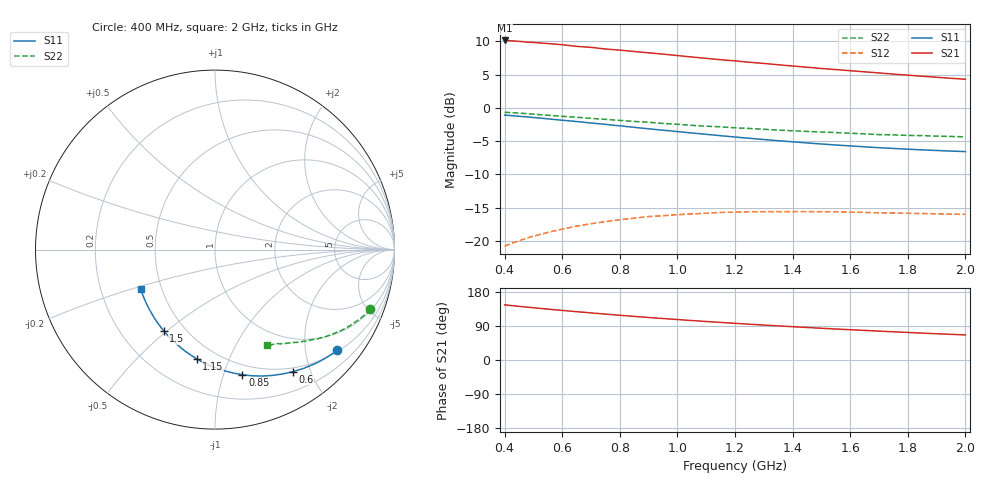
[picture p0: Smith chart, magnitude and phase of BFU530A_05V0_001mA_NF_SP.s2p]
! Filename:  P:\Prog\Test\Noise\ATS_data\Testdata_Net\06 Compressed Noise after Statistics\BFU530A_APG2013_33_A05_05p0V_001mA_SP_CM01_D.sf
! Date/Time: Tue 16/Apr/2013 15:10:54
! BFU530A_APG2013_33_A05_05p0V_1to25mA_NF_CM01_Bias1_R.sf
! Noise Parameter Data File
! BFU530A_APG2013_33_A05_05p0V_1to25mA_NF_CM01
! Date/time: Fri Apr 12 15:27:54 2013
! freq range =  0.4000 to  2.0000 GHz, 37 points
! bias range =  1.0000 to 25.0000 mA, 8 points
! bias supplies used: 1 1 0 0 0 0
! VAR bias_mode= 1  ! Specify V_out, I_out
! VAR bias_var = 1  ! Bias variable = I_out
! VAR V_out= 5.001000
! VAR I_out= 1.000000
! VAR V_in= 0.783300
! VAR I_in= 0.010301
! Device data file deembeded for feedlines and parallel
! Original file: \06 Compressed Noise after Statistics\BFU530A_APG2013_33_A05_05p0V_001mA_SP_CM01_R.sf
! Feed-files: PR017V01_150413_Feed1.s2p, PR017V01_150413_Feed2.s2p
! Parallel-file: PR017V01_150413_Par.s2p
# MHz S MA R 50
!  Freq-MHz  S11-mag  S11-arg  S21-mag  S21-arg  S12-mag  S12-arg  S22-mag  S22-arg
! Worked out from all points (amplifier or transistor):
!   37 points, 400 MHz to 2 GHz, reference 50 ohm
!   highest |S21| = 10.1 dB at 400 MHz (marker M1)
!   |S21| within 3 dB of that: start of sweep to 1.18 GHz
!   unconditionally stable (mu >= 1): nowhere
!   at 500 MHz: K = 0.23, MSG = 14.5 dB, |S12| = -19.3 dB
!   at 1.1 GHz: K = 0.48, MSG = 11.6 dB, |S12| = -15.8 dB
!   at 2 GHz: K = 0.88, MSG = 10.1 dB, |S12| = -16.0 dB
!   lowest NFmin = 0.41 dB at 433 MHz
!   S11 on the Smith chart (normalised r, x): 400 MHz: 0.53, -2.70; 600 MHz: 0.45, -1.74; 850 MHz: 0.41, -1.16; 1.15 GHz: 0.39, -0.77; 1.5 GHz: 0.38, -0.49; 2 GHz: 0.38, -0.22
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400  0.8821 -39.4  3.205 145.5  0.09142 65.2  0.9266 -20.9
420  0.8752 -41.4  3.193 143.8  0.0951 64.1  0.9205 -21.9
440  0.8679 -43.2  3.168 142.3  0.09865 63.0  0.915 -22.7
480  0.8538 -46.7  3.109 139.4  0.1054 61.0  0.9026 -24.5
500  0.8459 -48.6  3.097 137.9  0.1086 60.0  0.8965 -25.3
550  0.8265 -53.1  3.038 134.3  0.1159 57.6  0.8795 -27.4
600  0.8068 -57.4  2.979 130.8  0.1228 55.4  0.8639 -29.3
650  0.7891 -61.5  2.893 127.5  0.1293 53.3  0.8497 -31.0
700  0.7692 -65.8  2.845 124.2  0.1346 51.2  0.8335 -32.8
750  0.7516 -69.6  2.764 121.1  0.1399 49.4  0.8189 -34.4
800  0.7324 -73.7  2.712 118.1  0.1444 47.6  0.8044 -36.0
850  0.7136 -77.6  2.648 115.0  0.1484 45.9  0.7903 -37.5
950  0.6788 -85.2  2.531 109.4  0.1548 42.9  0.7632 -40.4
1050  0.6471 -92.3  2.408 104.1  0.1597 40.3  0.7386 -42.8
1150  0.6176 -99.4  2.299 99.2  0.1638 38.0  0.7197 -45.1
1200  0.6035 -102.8  2.25 96.8  0.1644 37.0  0.7077 -46.3
1350  0.5663 -112.7  2.106 90.0  0.166 34.7  0.6799 -49.5
1500  0.5351 -122.3  1.975 83.8  0.166 33.0  0.6579 -52.5
1650  0.5094 -131.5  1.864 78.1  0.1639 32.5  0.6378 -55.4
1750  0.4955 -137.5  1.792 74.4  0.1623 32.6  0.626 -57.1
1850  0.4834 -143.2  1.728 71.0  0.1608 33.0  0.6182 -59.0
2000  0.4692 -151.8  1.638 66.1  0.1584 34.6  0.6052 -61.7
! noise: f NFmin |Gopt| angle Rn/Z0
400  0.453  0.7259  22.92  0.3355
460  0.4897  0.7062  27.72  0.354
600  0.5741  0.6746  35.72  0.3269
800  0.5872  0.6135  51.16  0.2615
1000  0.6876  0.588  63.33  0.2405
1200  0.7661  0.5932  74.17  0.2379
1400  0.7937  0.5676  89.47  0.1855
1600  0.8718  0.5618  101.7  0.1471
1800  0.7061  0.5259  123.1  0.0959
2000  0.8508  0.5969  130.3  0.0784
